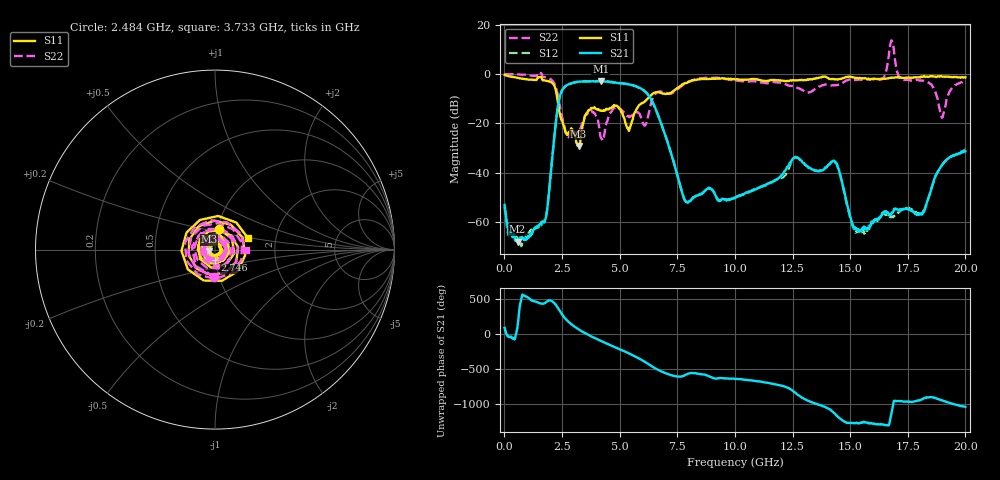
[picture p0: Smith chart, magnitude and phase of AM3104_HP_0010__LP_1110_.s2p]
!Created with skrf (http://scikit-rf.org).
# Hz S RI R 50.0
!freq ReS11 ImS11 ReS21 ImS21 ReS12 ImS12 ReS22 ImS22
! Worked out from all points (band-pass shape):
!   1601 points, 10 MHz to 20 GHz, reference 50 ohm
!   highest |S21| = -2.86 dB at 4.183 GHz (marker M1); lowest = -67.9 dB at 572.2 MHz (marker M2)
!   |S21| within 3 dB of the highest: 2.553 GHz to 5.918 GHz (3.365 GHz wide, 79.5 % of centre)
!   lowest |S11| = -29.2 dB at 3.221 GHz (marker M3), VSWR 1.07, Z = 46.8 - j0.962 ohm
!   |S11| at or under -10 dB: 2.299 GHz to 6.215 GHz (3.916 GHz wide, 92 % of centre)
!   |S22| runs from -26.9 to 13.6 dB; largest |S21 - S12| = 0.077
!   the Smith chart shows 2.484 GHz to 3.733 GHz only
!   S11 on the Smith chart (normalised r, x): 2.484 GHz: 1.02, +0.23; 2.746 GHz: 0.99, -0.12; 3.733 GHz: 1.44, +0.19
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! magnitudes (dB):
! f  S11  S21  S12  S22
! 10 MHz  -0.4  -53.0  -53.7  0.0
! 572.2 MHz  -1.5  -67.9  -67.2  -0.1
! 1.772 GHz  -2.7  -59.0  -58.6  -1.2
! 2.484 GHz  -18.8  -6.9  -7.0  -16.5
! 2.746 GHz  -24.5  -4.3  -4.4  -25.1
! 3.221 GHz  -29.2  -3.1  -3.2  -24.1
! 3.346 GHz  -23.6  -3.0  -3.1  -20.8
! 3.733 GHz  -14.2  -2.9  -3.0  -15.3
! 4.183 GHz  -14.9  -2.9  -2.9  -25.7
! 5.395 GHz  -23.0  -4.2  -4.2  -17.4
! 6.107 GHz  -11.0  -7.1  -7.1  -20.8
! 6.682 GHz  -7.3  -17.0  -17.1  -7.1
! 7.881 GHz  -3.7  -51.6  -51.9  -3.6
! 10.01 GHz  -2.2  -50.3  -50.1  -2.7
! 13.34 GHz  -2.2  -38.6  -38.7  -7.0
! 14.38 GHz  -2.1  -35.8  -36.1  -4.5
! 15.25 GHz  -1.6  -62.5  -64.2  -2.4
! 16.39 GHz  -1.9  -56.9  -56.5  -2.0
! 16.68 GHz  -1.7  -56.8  -57.8  7.3
! 18.13 GHz  -1.1  -56.9  -55.8  -2.7
! 18.98 GHz  -1.0  -37.0  -37.1  -17.6
! 20 GHz  -1.3  -31.3  -30.7  -2.9
